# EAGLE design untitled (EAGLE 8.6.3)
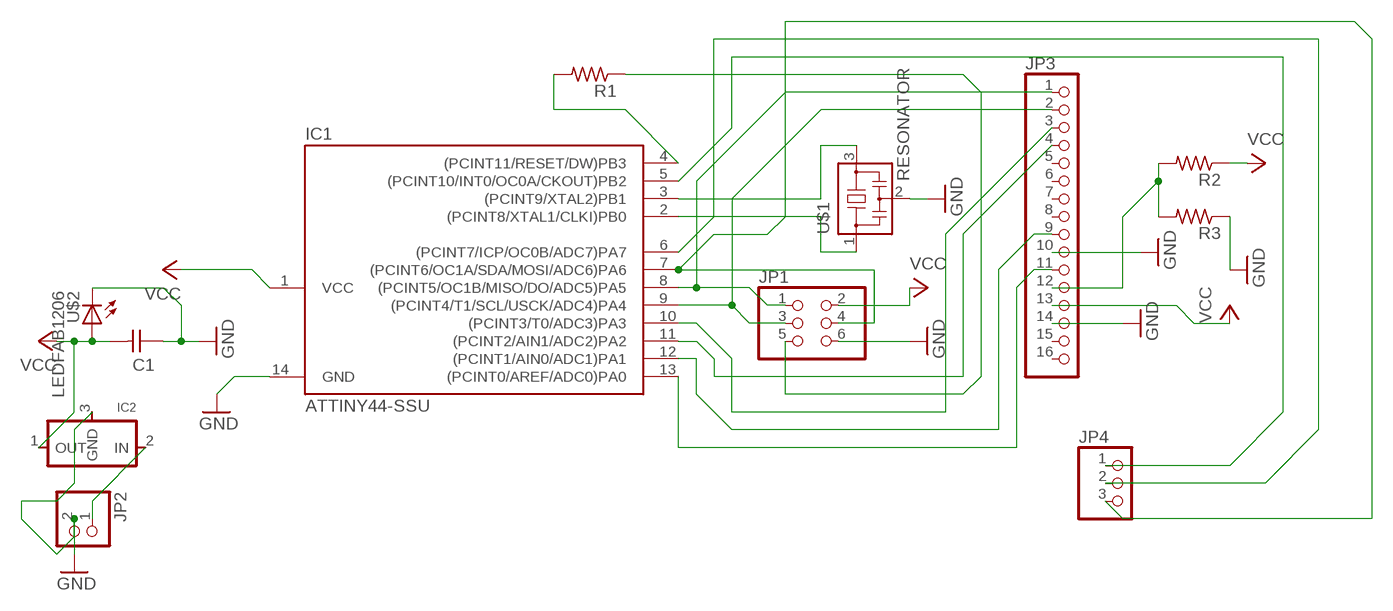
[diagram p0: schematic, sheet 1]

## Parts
C1  CAP-UNPOLARIZEDFAB  [C1206FAB]
IC1  ATTINY44-SSU  [SOIC14]
IC2  REGULATORSOT23  [SOT23]
JP1  PINHD-2X3-SMD  [2X03SMD]
JP2  PINHD-1X2  [1X02]
JP3  PINHD-1X16  [1X16]
JP4  PINHD-1X3  [1X03]
R1  RES-US1206FAB  [R1206FAB]
R2  RES-US1206FAB  [R1206FAB]
R3  RES-US1206FAB  [R1206FAB]
U$1  RESONATOR  [EFOBM]
U$2  LEDFAB1206  [LED1206FAB]

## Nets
GND: C1.1 IC1.14(GND) IC2.3(GND) JP1.6 JP2.2 JP3.10 JP3.14 R3.1 U$1.2 U$2.2(C)
N$1: IC1.3((PCINT9/XTAL2)PB1) U$1.3
N$2: IC1.2((PCINT8/XTAL1/CLKI)PB0) U$1.1
N$3: IC1.7((PCINT6/OC1A/SDA/MOSI/ADC6)PA6) JP1.4 JP4.3
N$4: IC1.8((PCINT5/OC1B/MISO/DO/ADC5)PA5) JP1.1 JP3.1
N$5: IC1.9((PCINT4/T1/SCL/USCK/ADC4)PA4) JP1.3 JP3.2
N$6: IC1.11((PCINT2/AIN1/ADC2)PA2) JP3.4
N$7: JP3.12 R2.2 R3.2
N$8: IC1.4((PCINT11/RESET/DW)PB3) R1.2
N$9: JP1.5 R1.1
N$10: IC1.5((PCINT10/INT0/OC0A/CKOUT)PB2) JP4.1
N$11: IC1.10((PCINT3/T0/ADC3)PA3) JP3.3
N$12: IC1.13((PCINT0/AREF/ADC0)PA0) JP3.11
N$13: IC1.12((PCINT1/AIN0/ADC1)PA1) JP3.9
N$14: IC1.6((PCINT7/ICP/OC0B/ADC7)PA7) JP4.2
N$17: IC2.2(IN) JP2.1
VCC: C1.2 IC1.1(VCC) IC2.1(OUT) JP1.2 JP3.13 R2.1 U$2.1(A)
Unconnected: JP3.5 JP3.6 JP3.7 JP3.8 JP3.15 JP3.16

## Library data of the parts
C1 = fab:CAP-UNPOLARIZED
IC1 = fab:ATTINY44
IC2 = fab:REGULATOR
JP1 = fab:PINHD-2X3-SMD: PIN HEADER
JP2 = pinhead:PINHD-1X2: PIN HEADER
JP3 = pinhead:PINHD-1X16: PIN HEADER
JP4 = pinhead:PINHD-1X3: PIN HEADER
R1-R3 = fab:RES-US: Resistor (US Symbol)
U$1 = fab:RESONATOR
U$2 = fab:LED: LED

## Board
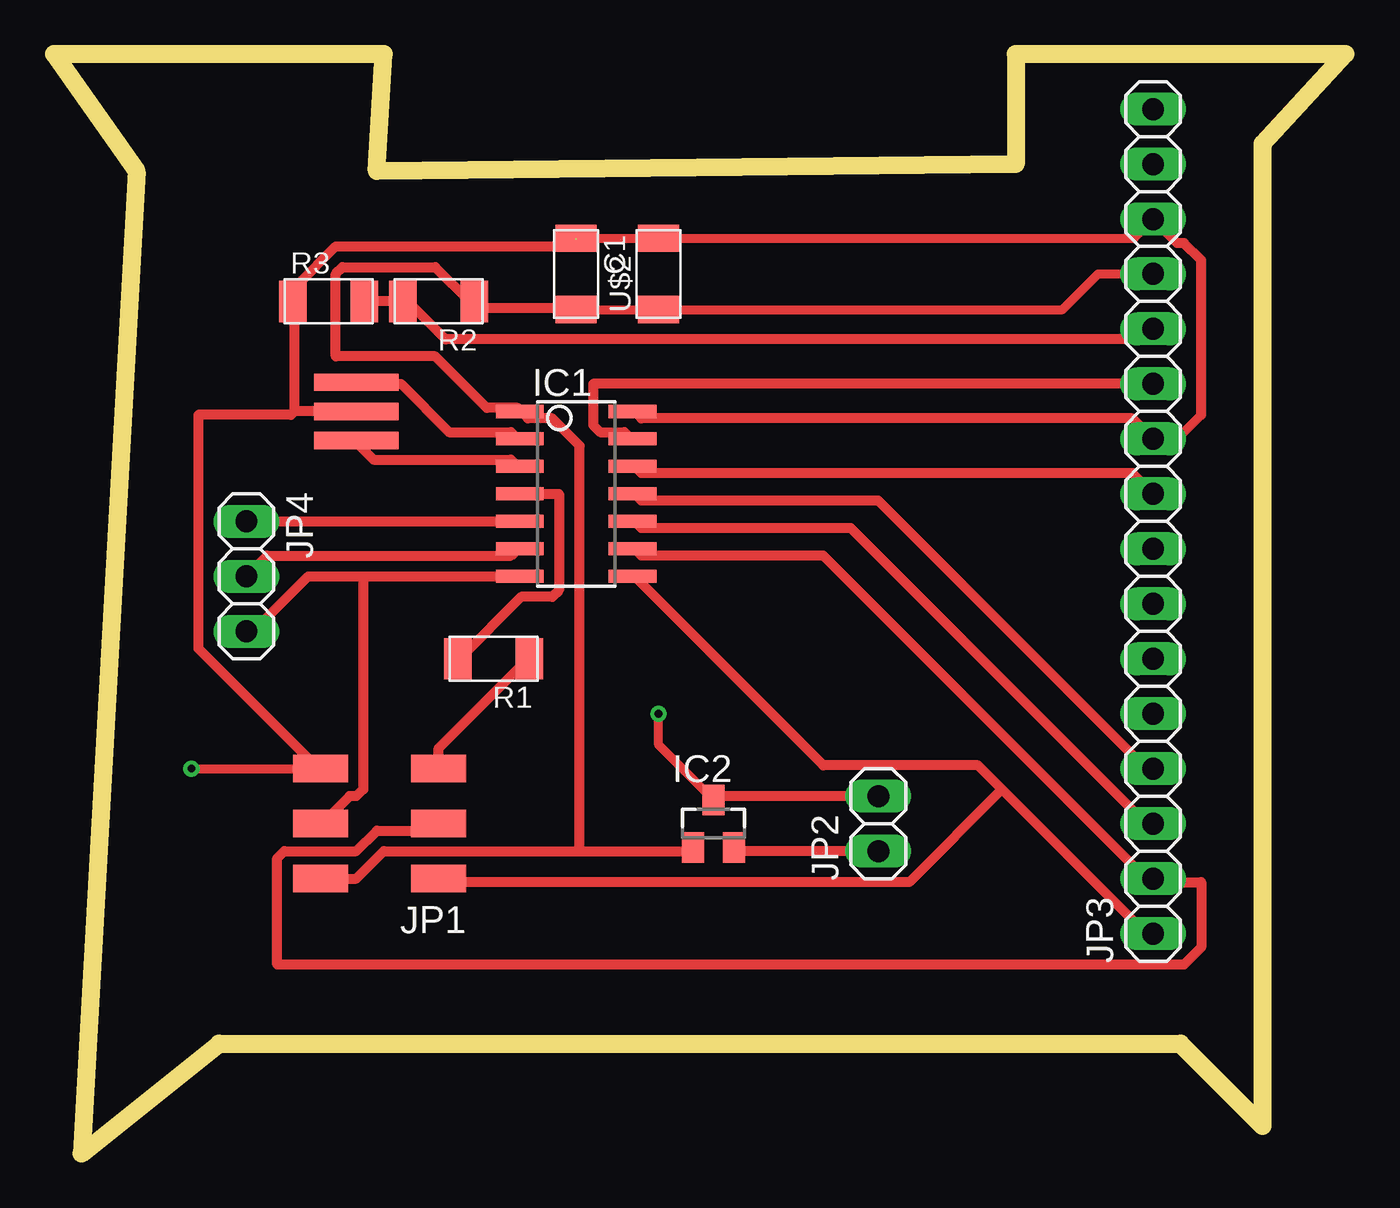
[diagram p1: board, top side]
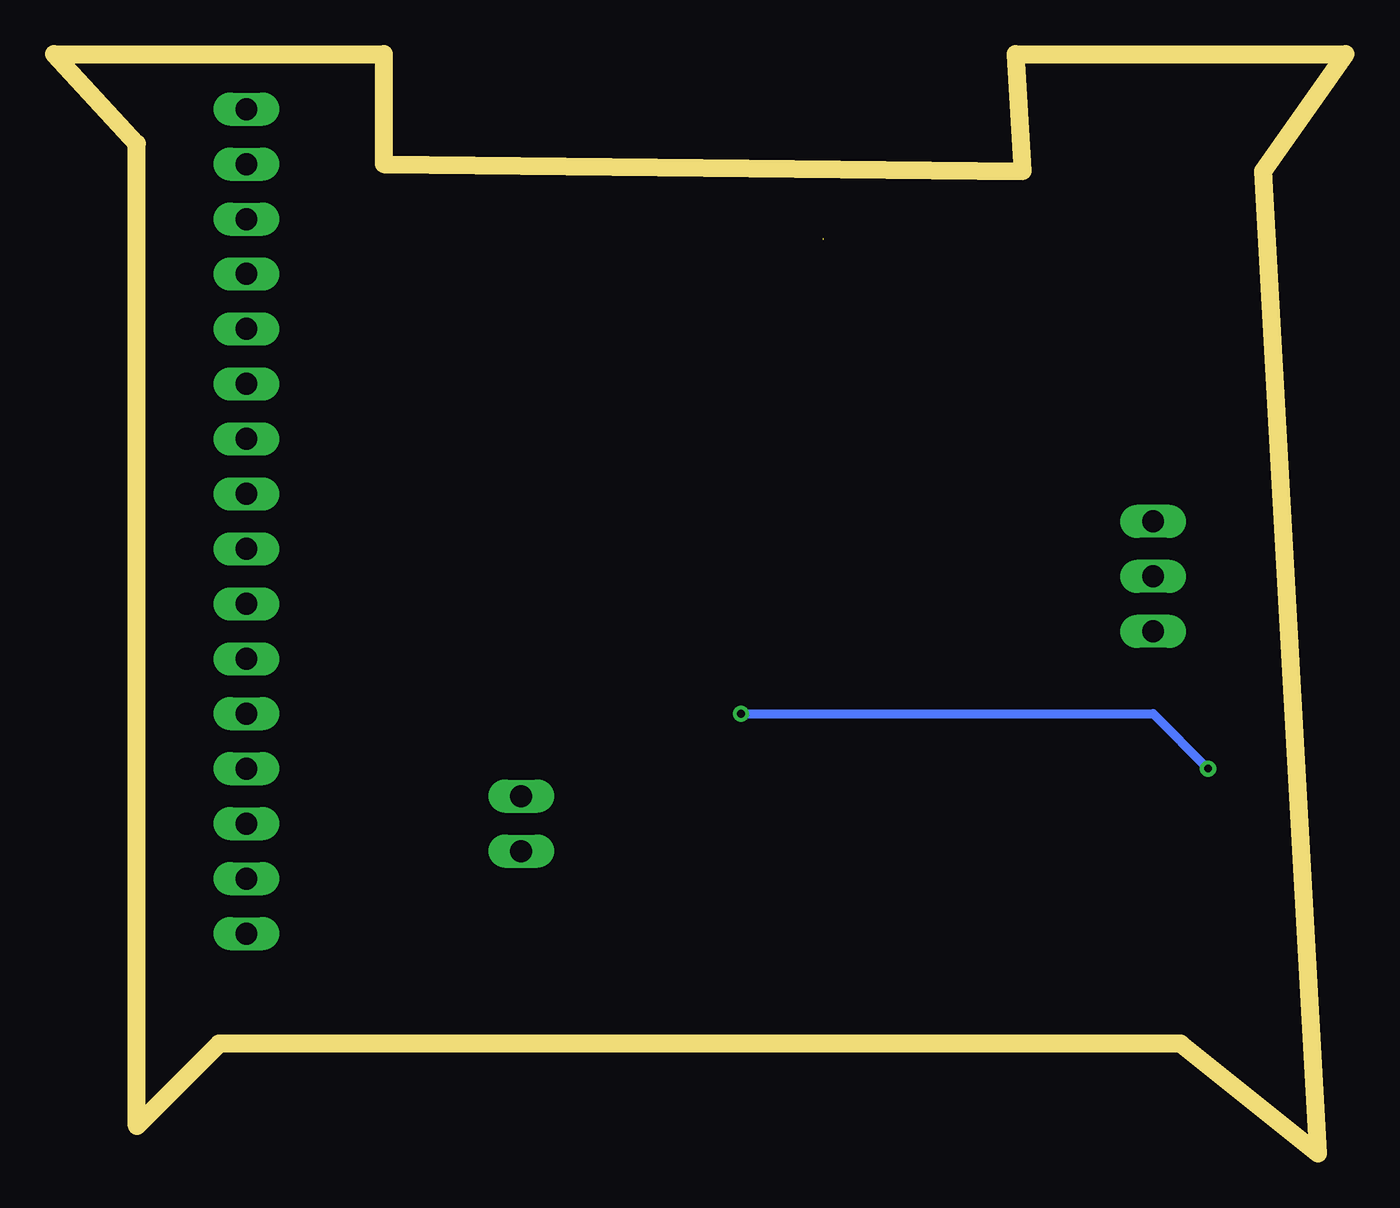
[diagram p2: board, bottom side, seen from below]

Size 59.69 x 50.8 mm. Coordinates in mm from the lower left corner, seen from the top.
Outline: 1.27,0 7.62,5.08 52.07,5.08 55.86,1.27 55.86,46.66 59.69,50.8 44.45,50.8 44.45,45.72 14.91,45.39 15.24,50.8 0,50.8 3.81,45.39 1.27,0
Copper layers (1*16): Top 0.035mm / dielectric 1.5mm / Bottom 0.035mm
Design rules "default *": minimum track width 18mil, minimum drill 0.35mm, track to track 16mil, track to pad 16mil, pad to pad 16mil, via to via 16mil, smd to smd 16mil, copper to edge 40mil, drill to drill 6mil, minimum pad ring 10mil, minimum via ring 8mil, stop-mask expansion 4mil, vias tented up to drill 0mil, thermal gap 10mil

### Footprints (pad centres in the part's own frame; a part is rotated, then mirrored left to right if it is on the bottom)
C1206FAB = smd 1.27 x 1.905: 1 -1.651,0; 2 1.651,0
SOIC14 = smd 0.61 x 2.21: 1 -3.81,-2.603; 2 -2.54,-2.603; 3 -1.27,-2.603; 4 0,-2.603; 5 1.27,-2.603; 6 2.54,-2.603; 7 3.81,-2.603; 8 3.81,2.603; 9 2.54,2.603; 10 1.27,2.603; 11 0,2.603; 12 -1.27,2.603; 13 -2.54,2.603; 14 -3.81,2.603
SOT23 = smd 1 x 1.4: 1 -0.95,-1.1; 2 0.95,-1.1; 3 0,1.1
2X03SMD = smd 2.54 x 1.27: 1 -2.54,2.54; 2 2.92,2.54; 3 -2.54,0; 4 2.92,0; 5 -2.54,-2.54; 6 2.92,-2.54
1X02 = drill 1.016 long: 1 -1.27,0; 2 1.27,0
1X16 = drill 1.016 long: 1 -19.05,0; 2 -16.51,0; 3 -13.97,0; 4 -11.43,0; 5 -8.89,0; 6 -6.35,0; 7 -3.81,0; 8 -1.27,0; 9 1.27,0; 10 3.81,0; 11 6.35,0; 12 8.89,0; 13 11.43,0; 14 13.97,0; 15 16.51,0; 16 19.05,0
1X03 = drill 1.016 long: 1 -2.54,0; 2 0,0; 3 2.54,0
R1206FAB = smd 1.27 x 1.905: 1 -1.651,0; 2 1.651,0
EFOBM = smd 0.8 x 3.9: 1 -1.35,0; 2 0,0; 3 1.35,0
LED1206FAB = smd 1.27 x 1.905: 1 -1.651,0; 2 1.651,0

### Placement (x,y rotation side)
C1  24.13,40.64 270 top
IC1  24.13,30.48 270 top
IC2  30.48,15.24 0 top
JP1  15.24,15.24 180 top
JP2  38.1,15.24 90 top
JP3  50.8,29.21 90 top
JP4  8.89,26.67 270 top
R1  20.32,22.86 180 top
R2  17.78,39.37 180 top
R3  12.7,39.37 0 top
U$1  13.97,34.29 270 top
U$2  27.94,40.64 90 top

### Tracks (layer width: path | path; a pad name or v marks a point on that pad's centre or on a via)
GND  (via drill 0.35)  (1 unrouted)
  Top 0.406: JP3.14 49.91,42.29 U$2.2 C1.1 | JP3.10 51.91,33.02 53.02,34.13 | IC2.3 27.94,18.88 v27.94,20.32 | v6.35,17.78 12.22,17.78
  Top 0.457: JP3.10 49.85,33.97 27.15,33.97 26.83,34.29 IC1.14 | JP3.14 51.91,42.07 52.23,42.07 53.02,41.27 53.02,34.13 | 11.11,34.29 11.11,39.37 R3.1 11.27,39.53 11.27,40.16 13.02,41.91 23.81,41.91 24.13,42.23 | U$1.2 11.11,34.29 | JP1.6 12.22,17.78 6.67,23.34 6.67,34.13 10.95,34.13 11.11,34.29 | 24.29,42.39 C1.1 | JP2.2 30.64,16.51 IC2.3
  Bottom 0.406: v27.94,20.32 8.89,20.32 v6.35,17.78
N$1
  Top 0.457: IC1.3 21.43,31.75 21.11,32.07 14.76,32.07 13.97,32.86 U$1.3
N$2
  Top 0.457: IC1.2 21.43,33.02 21.11,33.34 18.26,33.34 16.03,35.56 13.97,35.56 U$1.1
N$3
  Top 0.457: 14.29,26.67 11.75,26.67 9.21,24.13 JP4.3 | 14.29,26.67 IC1.7 | 14.29,26.67 14.29,16.83 13.97,16.51 13.65,16.51 12.38,15.24 JP1.4
N$4
  Top 0.457: 43.81,16.83 50.48,10.16 JP3.1 | 43.81,16.83 42.7,17.94 35.56,17.94 26.83,26.67 IC1.8 | JP1.1 17.94,12.54 39.53,12.54 43.81,16.83
N$5
  Top 0.457: IC1.9 26.83,27.94 27.15,27.62 35.56,27.62 50.48,12.7 JP3.2 50.96,12.54 53.02,12.54 53.02,9.52 52.23,8.73 10.32,8.73 10.32,13.65 10.64,13.97 13.97,13.97 14.92,14.92 17.46,14.92 JP1.3
N$6
  Top 0.457: JP3.4 50.48,17.78 38.1,30.16 27.15,30.16 26.83,30.48 IC1.11
N$7
  Top 0.457: R3.2 R2.2 16.35,39.37 18.1,37.62 50.32,37.62 JP3.12
N$8
  Top 0.457: IC1.4 23.34,30.48 23.34,26.03 23.02,25.72 21.59,25.72 18.73,22.86 R1.2
N$9
  Top 0.457: JP1.5 17.78,18.73 21.91,22.86 R1.1
N$10
  Top 0.457: JP4.1 IC1.5
N$11
  Top 0.457: JP3.3 50.48,15.24 36.83,28.89 27.15,28.89 26.83,29.21 IC1.10
N$12
  Top 0.457: JP3.11 24.92,35.56 24.92,33.66 25.24,33.34 26.35,33.34 26.67,33.02 IC1.13
N$13
  Top 0.457: JP3.9 49.85,31.43 27.15,31.43 26.83,31.75 IC1.12
N$14
  Top 0.457: JP4.2 9.84,27.62 21.11,27.62 21.43,27.94 IC1.6
N$17
  Top 0.457: JP2.1 31.59,13.97 IC2.2
VCC
  Top 0.406: JP3.13 48.26,40.64 46.61,38.99 U$2.1 C1.2
  Top 0.457: 24.29,39.21 C1.2 24.13,39.05 19.84,39.05 19.53,39.37 R2.1 19.21,39.37 17.62,40.96 13.34,40.96 13.02,40.64 13.02,36.83 17.62,36.83 20,34.45 21.43,34.45 IC1.1 21.59,34.29 21.91,33.97 23.02,33.97 24.29,32.7 24.29,13.97 | 24.29,13.97 15.24,13.97 13.97,12.7 JP1.2 | 24.29,13.97 29.37,13.97 IC2.1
